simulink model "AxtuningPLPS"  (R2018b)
settings: Solver=VariableStepAuto  StartTime=0.0  StopTime=1  RelTol=1e-3
libraries: fuzblock x18

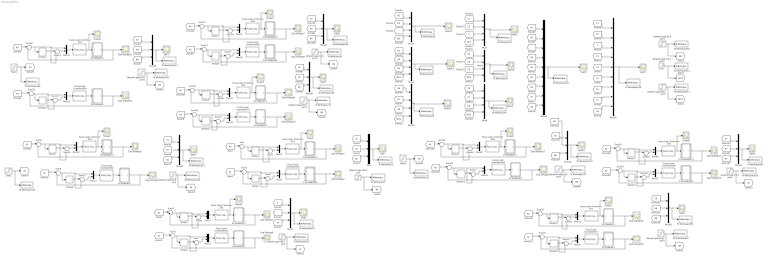
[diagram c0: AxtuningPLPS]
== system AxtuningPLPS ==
  2V EDMGAP 1 : Subsystem
  2V EDMGAP 2 : Subsystem
  2V EDMGAP 3 : Subsystem
  2V EDMGAP1 : Subsystem
  2V EDMGAP2 : Subsystem
  2V EDMGAP3 : Subsystem
  3.5V EDMGAP 1 : Subsystem
  3.5V EDMGAP 2 : Subsystem
  3.5V EDMGAP 3 : Subsystem
  3.5V EDMGAP1 : Subsystem
  3.5V EDMGAP2 : Subsystem
  3.5V EDMGAP3 : Subsystem
  5V EDMGAP 1 : Subsystem
  5V EDMGAP 2 : Subsystem
  5V EDMGAP 3 : Subsystem
  5V EDMGAP1 : Subsystem
  5V EDMGAP2 : Subsystem
  5V EDMGAP3 : Subsystem
  Delay{1..18} (18 alike) : Delay  DelayLength=1
  Fuzzy Logic Controller 3X1 : fuzblock/Fuzzy Logic  Controller  FIS=PL36  OutputSampleNumber=101  DataType=double  FuzzifiedInputs=off  RuleFiringStrengths=off  RuleOutputs=off  AggregatedOutputs=off  SimulateUsing=Interpreted execution  OutOfRangeInputValueMessage=warning  NoRuleFiredMessage=warning  EmptyOutputFuzzySetMessage=warning
  Fuzzy Logic Controller 3X2 : fuzblock/Fuzzy Logic  Controller  FIS=PL60  OutputSampleNumber=101  DataType=double  FuzzifiedInputs=off  RuleFiringStrengths=off  RuleOutputs=off  AggregatedOutputs=off  SimulateUsing=Interpreted execution  OutOfRangeInputValueMessage=warning  NoRuleFiredMessage=warning  EmptyOutputFuzzySetMessage=warning
  Fuzzy Logic Controller 3X3 : fuzblock/Fuzzy Logic  Controller  FIS=PL40  OutputSampleNumber=101  DataType=double  FuzzifiedInputs=off  RuleFiringStrengths=off  RuleOutputs=off  AggregatedOutputs=off  SimulateUsing=Interpreted execution  OutOfRangeInputValueMessage=warning  NoRuleFiredMessage=warning  EmptyOutputFuzzySetMessage=warning
  Fuzzy Logic Controller 3X4 : fuzblock/Fuzzy Logic  Controller  FIS=PL36  OutputSampleNumber=101  DataType=double  FuzzifiedInputs=off  RuleFiringStrengths=off  RuleOutputs=off  AggregatedOutputs=off  SimulateUsing=Interpreted execution  OutOfRangeInputValueMessage=warning  NoRuleFiredMessage=warning  EmptyOutputFuzzySetMessage=warning
  Fuzzy Logic Controller 3X5 : fuzblock/Fuzzy Logic  Controller  FIS=PL60  OutputSampleNumber=101  DataType=double  FuzzifiedInputs=off  RuleFiringStrengths=off  RuleOutputs=off  AggregatedOutputs=off  SimulateUsing=Interpreted execution  OutOfRangeInputValueMessage=warning  NoRuleFiredMessage=warning  EmptyOutputFuzzySetMessage=warning
  Fuzzy Logic Controller 3X6 : fuzblock/Fuzzy Logic  Controller  FIS=PL40  OutputSampleNumber=101  DataType=double  FuzzifiedInputs=off  RuleFiringStrengths=off  RuleOutputs=off  AggregatedOutputs=off  SimulateUsing=Interpreted execution  OutOfRangeInputValueMessage=warning  NoRuleFiredMessage=warning  EmptyOutputFuzzySetMessage=warning
  Fuzzy Logic Controller 3X7 : fuzblock/Fuzzy Logic  Controller  FIS=PL36  OutputSampleNumber=101  DataType=double  FuzzifiedInputs=off  RuleFiringStrengths=off  RuleOutputs=off  AggregatedOutputs=off  SimulateUsing=Interpreted execution  OutOfRangeInputValueMessage=warning  NoRuleFiredMessage=warning  EmptyOutputFuzzySetMessage=warning
  Fuzzy Logic Controller 3X8 : fuzblock/Fuzzy Logic  Controller  FIS=PL60  OutputSampleNumber=101  DataType=double  FuzzifiedInputs=off  RuleFiringStrengths=off  RuleOutputs=off  AggregatedOutputs=off  SimulateUsing=Interpreted execution  OutOfRangeInputValueMessage=warning  NoRuleFiredMessage=warning  EmptyOutputFuzzySetMessage=warning
  Fuzzy Logic Controller 3X9 : fuzblock/Fuzzy Logic  Controller  FIS=PL40  OutputSampleNumber=101  DataType=double  FuzzifiedInputs=off  RuleFiringStrengths=off  RuleOutputs=off  AggregatedOutputs=off  SimulateUsing=Interpreted execution  OutOfRangeInputValueMessage=warning  NoRuleFiredMessage=warning  EmptyOutputFuzzySetMessage=warning
  Fuzzy Logic Controller5X1 : fuzblock/Fuzzy Logic  Controller  FIS=PS25  OutputSampleNumber=101  DataType=double  FuzzifiedInputs=off  RuleFiringStrengths=off  RuleOutputs=off  AggregatedOutputs=off  SimulateUsing=Interpreted execution  OutOfRangeInputValueMessage=warning  NoRuleFiredMessage=warning  EmptyOutputFuzzySetMessage=warning
  Fuzzy Logic Controller5X2 : fuzblock/Fuzzy Logic  Controller  FIS=PS39  OutputSampleNumber=101  DataType=double  FuzzifiedInputs=off  RuleFiringStrengths=off  RuleOutputs=off  AggregatedOutputs=off  SimulateUsing=Interpreted execution  OutOfRangeInputValueMessage=warning  NoRuleFiredMessage=warning  EmptyOutputFuzzySetMessage=warning
  Fuzzy Logic Controller5X3 : fuzblock/Fuzzy Logic  Controller  FIS=PS25  OutputSampleNumber=101  DataType=double  FuzzifiedInputs=off  RuleFiringStrengths=off  RuleOutputs=off  AggregatedOutputs=off  SimulateUsing=Interpreted execution  OutOfRangeInputValueMessage=warning  NoRuleFiredMessage=warning  EmptyOutputFuzzySetMessage=warning
  Fuzzy Logic Controller5X4 : fuzblock/Fuzzy Logic  Controller  FIS=PS39  OutputSampleNumber=101  DataType=double  FuzzifiedInputs=off  RuleFiringStrengths=off  RuleOutputs=off  AggregatedOutputs=off  SimulateUsing=Interpreted execution  OutOfRangeInputValueMessage=warning  NoRuleFiredMessage=warning  EmptyOutputFuzzySetMessage=warning
  Fuzzy Logic Controller5X5 : fuzblock/Fuzzy Logic  Controller  FIS=PS35  OutputSampleNumber=101  DataType=double  FuzzifiedInputs=off  RuleFiringStrengths=off  RuleOutputs=off  AggregatedOutputs=off  SimulateUsing=Interpreted execution  OutOfRangeInputValueMessage=warning  NoRuleFiredMessage=warning  EmptyOutputFuzzySetMessage=warning
  Fuzzy Logic Controller5X6 : fuzblock/Fuzzy Logic  Controller  FIS=PS35  OutputSampleNumber=101  DataType=double  FuzzifiedInputs=off  RuleFiringStrengths=off  RuleOutputs=off  AggregatedOutputs=off  SimulateUsing=Interpreted execution  OutOfRangeInputValueMessage=warning  NoRuleFiredMessage=warning  EmptyOutputFuzzySetMessage=warning
  Fuzzy Logic Controller5X7 : fuzblock/Fuzzy Logic  Controller  FIS=PS25  OutputSampleNumber=101  DataType=double  FuzzifiedInputs=off  RuleFiringStrengths=off  RuleOutputs=off  AggregatedOutputs=off  SimulateUsing=Interpreted execution  OutOfRangeInputValueMessage=warning  NoRuleFiredMessage=warning  EmptyOutputFuzzySetMessage=warning
  Fuzzy Logic Controller5X8 : fuzblock/Fuzzy Logic  Controller  FIS=PS39  OutputSampleNumber=101  DataType=double  FuzzifiedInputs=off  RuleFiringStrengths=off  RuleOutputs=off  AggregatedOutputs=off  SimulateUsing=Interpreted execution  OutOfRangeInputValueMessage=warning  NoRuleFiredMessage=warning  EmptyOutputFuzzySetMessage=warning
  Fuzzy Logic Controller5X9 : fuzblock/Fuzzy Logic  Controller  FIS=PS35  OutputSampleNumber=101  DataType=double  FuzzifiedInputs=off  RuleFiringStrengths=off  RuleOutputs=off  AggregatedOutputs=off  SimulateUsing=Interpreted execution  OutOfRangeInputValueMessage=warning  NoRuleFiredMessage=warning  EmptyOutputFuzzySetMessage=warning
  GAP{,1..16} (17 alike) : Scope
  Gap Voltage{1..18} (18 alike) : Scope
  Mux{,6,12,26,30,40,44,48,58} (9 alike) : Mux  Inputs=3
  Mux{1,5,7,11,13,17,27,29,31,35,39,41,45,47,49,53,57,59} (18 alike) : Mux  Inputs=2
  Mux{2..4,8..10} (6 alike) : Mux
  Mux18 : Mux  Inputs=9
  Mux22 : Mux  Inputs=9
  Scope{,1..8} (9 alike) : Scope
  Setpoint gap (59,3 µm){,1..3} (4 alike) : Step  Time=0  After=59.3  SampleTime=0
  Setpoint gap (84,7 µm){,1..3} (4 alike) : Step  Time=0  After=84.7  SampleTime=0
  Setpoint gap(33,8 µm){,1..3} (4 alike) : Step  Time=0  After=33.8  SampleTime=0
  Step1 : Step  Time=0  After=3.5  SampleTime=0
  Step2 : Step  Time=0  After=2  SampleTime=0
  Step3 : Step  Time=0  After=5  SampleTime=0
  Sum{,1..35} (36 alike) : Sum  Inputs=|-+
  To Workspace1 : ToWorkspace  VariableName=setpointgap  SaveFormat=Timeseries  SampleTime=-1
  To Workspace10 : ToWorkspace  VariableName=setpointgap9  SaveFormat=Timeseries  SampleTime=-1
  To Workspace11 : ToWorkspace  VariableName=setpointgap10  SaveFormat=Timeseries  SampleTime=-1
  To Workspace12 : ToWorkspace  VariableName=setpointgap1  SaveFormat=Timeseries  SampleTime=-1
  To Workspace13 : ToWorkspace  VariableName=setpointgap11  SaveFormat=Timeseries  SampleTime=-1
  To Workspace15 : ToWorkspace  VariableName=setpointgap3  SaveFormat=Timeseries  SampleTime=-1
  To Workspace2 : ToWorkspace  VariableName=setpointgap4  SaveFormat=Timeseries  SampleTime=-1
  To Workspace22 : ToWorkspace  VariableName=gap10  SaveFormat=Timeseries  SampleTime=-1
  To Workspace23 : ToWorkspace  VariableName=setpointgap2  SaveFormat=Timeseries  SampleTime=-1
  To Workspace28 : ToWorkspace  VariableName=setpoint2  SaveFormat=Timeseries  SampleTime=-1
  To Workspace3 : ToWorkspace  VariableName=gap  SaveFormat=Timeseries  SampleTime=-1
  To Workspace33 : ToWorkspace  VariableName=gap1  SaveFormat=Timeseries  SampleTime=-1
  To Workspace39 : ToWorkspace  VariableName=gap18  SaveFormat=Timeseries  SampleTime=-1
  To Workspace4 : ToWorkspace  VariableName=gap2  SaveFormat=Timeseries  SampleTime=-1
  To Workspace43 : ToWorkspace  VariableName=gap19  SaveFormat=Timeseries  SampleTime=-1
  To Workspace44 : ToWorkspace  VariableName=gap11  SaveFormat=Timeseries  SampleTime=-1
  To Workspace45 : ToWorkspace  VariableName=setpointgap5  SaveFormat=Timeseries  SampleTime=-1
  To Workspace48 : ToWorkspace  VariableName=setpoint  SaveFormat=Timeseries  SampleTime=-1
  To Workspace5 : ToWorkspace  VariableName=gap3  SaveFormat=Timeseries  SampleTime=-1
  To Workspace53 : ToWorkspace  VariableName=gap12  SaveFormat=Timeseries  SampleTime=-1
  To Workspace58 : ToWorkspace  VariableName=gap13  SaveFormat=Timeseries  SampleTime=-1
  To Workspace59 : ToWorkspace  VariableName=setpointgap6  SaveFormat=Timeseries  SampleTime=-1
  To Workspace6 : ToWorkspace  VariableName=gap4  SaveFormat=Timeseries  SampleTime=-1
  To Workspace62 : ToWorkspace  VariableName=setpointgap7  SaveFormat=Timeseries  SampleTime=-1
  To Workspace69 : ToWorkspace  VariableName=gap14  SaveFormat=Timeseries  SampleTime=-1
  To Workspace7 : ToWorkspace  VariableName=gap5  SaveFormat=Timeseries  SampleTime=-1
  To Workspace70 : ToWorkspace  VariableName=setpointgap8  SaveFormat=Timeseries  SampleTime=-1
  To Workspace73 : ToWorkspace  VariableName=setpoint1  SaveFormat=Timeseries  SampleTime=-1
  To Workspace78 : ToWorkspace  VariableName=gap15  SaveFormat=Timeseries  SampleTime=-1
  To Workspace8 : ToWorkspace  VariableName=gap6  SaveFormat=Timeseries  SampleTime=-1
  To Workspace83 : ToWorkspace  VariableName=gap16  SaveFormat=Timeseries  SampleTime=-1
  To Workspace9 : ToWorkspace  VariableName=gap9  SaveFormat=Timeseries  SampleTime=-1
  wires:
  [N2] -> Mux/3
  Sum2/1 -> Mux1/2
  Mux5/1 -> Fuzzy Logic Controller5X5/1
  Delay2/1 -> Sum3/1
  [H2] -> Mux/2
  Mux/1 -> To Workspace9/1, GAP/1
  Sum/1 -> Delay1/1, Sum2/2, Mux1/1
  Delay1/1 -> Sum2/1
  Mux1/1 -> Fuzzy Logic Controller 3X3/1
  Fuzzy Logic Controller 3X3/1 -> Scope/1, 3.5V EDMGAP 1/1(In1)
  [A1] -> Sum1/1
  Sum1/1 -> Delay2/1, Sum3/2, Mux5/1
  Sum3/1 -> Mux5/2
  [C2] -> Mux/1
  [A1] -> Sum/1
  3.5V EDMGAP2/1(Out1) -> Gap Voltage2/1, Sum1/2
  3.5V EDMGAP 1/1(Out1) -> Sum/2, Gap Voltage1/1
  Fuzzy Logic Controller5X5/1 -> 3.5V EDMGAP2/1(In1)
  2V EDMGAP3/1(Out1) -> Gap Voltage6/1, Sum9/2
  Fuzzy Logic Controller5X2/1 -> 2V EDMGAP3/1(In1)
  [H1] -> Mux12/2
  [N1] -> Mux12/3
  [C1] -> Mux12/1
  Mux12/1 -> To Workspace33/1, GAP2/1
  Sum11/1 -> Mux17/2
  Sum9/1 -> Delay6/1, Sum11/2, Mux17/1
  Mux13/1 -> Fuzzy Logic Controller 3X2/1
  Step2/1 -> To Workspace28/1, [A1]
  [A1] -> Sum9/1
  Fuzzy Logic Controller 3X2/1 -> Scope2/1, 2V EDMGAP 3/1(In1)
  Delay5/1 -> Sum10/1
  2V EDMGAP 3/1(Out1) -> Sum8/2, Gap Voltage5/1
  Delay6/1 -> Sum11/1
  Sum10/1 -> Mux13/2
  [A1] -> Sum8/1
  Sum8/1 -> Delay5/1, Sum10/2, Mux13/1
  Mux17/1 -> Fuzzy Logic Controller5X2/1
  [H3] -> Mux30/2
  Fuzzy Logic Controller5X4/1 -> 2V EDMGAP1/1(In1)
  [N3] -> Mux30/3
  Sum17/1 -> Mux39/2
  Mux35/1 -> Fuzzy Logic Controller5X4/1
  [A3] -> Sum22/1
  Sum22/1 -> Delay11/1, Sum14/2, Mux31/1
  Step1/1 -> To Workspace48/1, [A3]
  3.5V EDMGAP1/1(Out1) -> Gap Voltage8/1, Sum13/2
  [A3] -> Sum13/1
  Fuzzy Logic Controller 3X6/1 -> Scope3/1, 3.5V EDMGAP 2/1(In1)
  Delay12/1 -> Sum15/1
  Fuzzy Logic Controller 3X5/1 -> Scope5/1, 2V EDMGAP 1/1(In1)
  [H4] -> Mux26/2
  [A3] -> Sum23/1
  Sum23/1 -> Delay12/1, Sum15/2, Mux35/1
  Mux26/1 -> To Workspace58/1, GAP5/1
  [C4] -> Mux26/1
  Mux30/1 -> To Workspace53/1, GAP7/1
  2V EDMGAP1/1(Out1) -> Gap Voltage12/1, Sum23/2
  Delay11/1 -> Sum14/1
  Sum15/1 -> Mux35/2
  Delay7/1 -> Sum16/1
  Fuzzy Logic Controller5X6/1 -> 3.5V EDMGAP1/1(In1)
  [A3] -> Sum12/1
  Delay8/1 -> Sum17/1
  Mux31/1 -> Fuzzy Logic Controller 3X5/1
  Mux27/1 -> Fuzzy Logic Controller 3X6/1
  3.5V EDMGAP 2/1(Out1) -> Sum12/2, Gap Voltage7/1
  [C3] -> Mux30/1
  Sum13/1 -> Delay8/1, Sum17/2, Mux39/1
  Sum12/1 -> Delay7/1, Sum16/2, Mux27/1
  2V EDMGAP 1/1(Out1) -> Sum22/2, Gap Voltage11/1
  Sum16/1 -> Mux27/2
  Sum14/1 -> Mux31/2
  [N4] -> Mux26/3
  Mux39/1 -> Fuzzy Logic Controller5X6/1
  Setpoint gap(33,8 µm)1/1 -> [N3], To Workspace45/1
  Setpoint gap (59,3 µm)1/1 -> [N4], To Workspace2/1
  Setpoint gap(33,8 µm)/1 -> [N1], To Workspace23/1
  Setpoint gap (59,3 µm)/1 -> [N2], To Workspace1/1
  Sum4/1 -> Delay3/1, Sum6/2, Mux7/1
  Mux7/1 -> Fuzzy Logic Controller 3X1/1
  Mux6/1 -> To Workspace22/1, GAP1/1
  5V EDMGAP1/1(Out1) -> Gap Voltage4/1, Sum5/2
  Setpoint gap (84,7 µm)/1 -> [N], To Workspace12/1
  5V EDMGAP 2/1(Out1) -> Sum4/2, Gap Voltage3/1
  Mux11/1 -> Fuzzy Logic Controller5X1/1
  Delay4/1 -> Sum7/1
  Fuzzy Logic Controller 3X1/1 -> Scope1/1, 5V EDMGAP 2/1(In1)
  Fuzzy Logic Controller5X1/1 -> 5V EDMGAP1/1(In1)
  Sum7/1 -> Mux11/2
  Sum6/1 -> Mux7/2
  Sum5/1 -> Delay4/1, Sum7/2, Mux11/1
  Delay3/1 -> Sum6/1
  [A1] -> Sum5/1
  [A1] -> Sum4/1
  [C] -> Mux6/1
  [H] -> Mux6/2
  [N] -> Mux6/3
  Setpoint gap (84,7 µm)1/1 -> [N5], To Workspace15/1
  Sum20/1 -> Mux41/2
  Sum19/1 -> Delay10/1, Sum21/2, Mux29/1
  [N5] -> Mux40/3
  Sum21/1 -> Mux29/2
  [A3] -> Sum19/1
  Delay9/1 -> Sum20/1
  Fuzzy Logic Controller5X3/1 -> 5V EDMGAP2/1(In1)
  Mux41/1 -> Fuzzy Logic Controller 3X4/1
  Delay10/1 -> Sum21/1
  Mux29/1 -> Fuzzy Logic Controller5X3/1
  5V EDMGAP2/1(Out1) -> Gap Voltage10/1, Sum19/2
  Mux40/1 -> To Workspace44/1, GAP6/1
  Fuzzy Logic Controller 3X4/1 -> Scope4/1, 5V EDMGAP 1/1(In1)
  Sum18/1 -> Delay9/1, Sum20/2, Mux41/1
  [A3] -> Sum18/1
  [H5] -> Mux40/2
  5V EDMGAP 1/1(Out1) -> Sum18/2, Gap Voltage9/1
  [C5] -> Mux40/1
  [H1] -> Mux22/1
  [H2] -> Mux22/2
  [C] -> Mux18/3
  [C2] -> Mux18/2
  [C1] -> Mux18/1
  [H] -> Mux22/3
  [C5] -> Mux18/6
  [C6] -> Mux18/7
  [C7] -> Mux18/8
  [C3] -> Mux18/4
  [C4] -> Mux18/5
  [C8] -> Mux18/9
  Mux18/1 -> To Workspace39/1, GAP3/1
  [H3] -> Mux22/4
  [H4] -> Mux22/5
  [H5] -> Mux22/6
  [H6] -> Mux22/7
  [H7] -> Mux22/8
  [H8] -> Mux22/9
  Mux22/1 -> To Workspace43/1, GAP4/1
  [C1] -> Mux2/1
  Mux2/1 -> To Workspace3/1, GAP11/1
  [C2] -> Mux2/2
  [C] -> Mux2/3
  [C4] -> Mux3/2
  [C3] -> Mux3/1
  Mux3/1 -> To Workspace4/1, GAP12/1
  [C5] -> Mux3/3
  [C8] -> Mux4/3
  [C7] -> Mux4/2
  Mux4/1 -> To Workspace5/1, GAP13/1
  [C6] -> Mux4/1
  Mux8/1 -> To Workspace6/1, GAP14/1
  [H] -> Mux8/3
  [H2] -> Mux8/2
  [H1] -> Mux8/1
  Mux9/1 -> To Workspace7/1, GAP15/1
  [H4] -> Mux9/2
  [H3] -> Mux9/1
  [H5] -> Mux9/3
  Mux10/1 -> To Workspace8/1, GAP16/1
  [H6] -> Mux10/1
  [H7] -> Mux10/2
  [H8] -> Mux10/3
  Fuzzy Logic Controller5X7/1 -> 5V EDMGAP3/1(In1)
  [C8] -> Mux58/1
  [H8] -> Mux58/2
  5V EDMGAP 3/1(Out1) -> Sum30/2, Gap Voltage15/1
  Mux59/1 -> Fuzzy Logic Controller 3X7/1
  [A2] -> Sum31/1
  Sum30/1 -> Delay15/1, Sum32/2, Mux59/1
  Setpoint gap (84,7 µm)2/1 -> [N8], To Workspace62/1
  5V EDMGAP3/1(Out1) -> Gap Voltage16/1, Sum31/2
  Sum32/1 -> Mux59/2
  Sum33/1 -> Mux47/2
  [A2] -> Sum30/1
  Sum31/1 -> Delay16/1, Sum33/2, Mux47/1
  [N8] -> Mux58/3
  2V EDMGAP 2/1(Out1) -> Sum34/2, Gap Voltage17/1
  Sum24/1 -> Delay13/1, Sum28/2, Mux45/1
  Delay15/1 -> Sum32/1
  [C6] -> Mux48/1
  3.5V EDMGAP 3/1(Out1) -> Sum24/2, Gap Voltage13/1
  Mux45/1 -> Fuzzy Logic Controller 3X9/1
  Fuzzy Logic Controller 3X7/1 -> Scope7/1, 5V EDMGAP 3/1(In1)
  [A2] -> Sum24/1
  Mux49/1 -> Fuzzy Logic Controller 3X8/1
  Delay14/1 -> Sum29/1
  Delay13/1 -> Sum28/1
  Fuzzy Logic Controller5X9/1 -> 3.5V EDMGAP3/1(In1)
  [C7] -> Mux44/1
  Mux48/1 -> To Workspace78/1, GAP10/1
  [H7] -> Mux44/2
  Fuzzy Logic Controller 3X8/1 -> Scope8/1, 2V EDMGAP 2/1(In1)
  Sum25/1 -> Delay14/1, Sum29/2, Mux57/1
  Fuzzy Logic Controller 3X9/1 -> Scope6/1, 3.5V EDMGAP 3/1(In1)
  [A2] -> Sum25/1
  Sum35/1 -> Delay18/1, Sum27/2, Mux53/1
  Mux44/1 -> To Workspace83/1, GAP8/1
  3.5V EDMGAP3/1(Out1) -> Gap Voltage14/1, Sum25/2
  Delay17/1 -> Sum26/1
  2V EDMGAP2/1(Out1) -> Gap Voltage18/1, Sum35/2
  Sum34/1 -> Delay17/1, Sum26/2, Mux49/1
  Mux53/1 -> Fuzzy Logic Controller5X8/1
  [H6] -> Mux48/2
  Sum29/1 -> Mux57/2
  Fuzzy Logic Controller5X8/1 -> 2V EDMGAP2/1(In1)
  [N7] -> Mux44/3
  [A2] -> Sum34/1
  Sum28/1 -> Mux45/2
  Sum26/1 -> Mux49/2
  [A2] -> Sum35/1
  Delay16/1 -> Sum33/1
  Mux47/1 -> Fuzzy Logic Controller5X7/1
  Step3/1 -> To Workspace73/1, [A2]
  Mux58/1 -> To Workspace69/1, GAP9/1
  Delay18/1 -> Sum27/1
  Sum27/1 -> Mux53/2
  [N6] -> Mux48/3
  Setpoint gap(33,8 µm)2/1 -> [N6], To Workspace70/1
  Mux57/1 -> Fuzzy Logic Controller5X9/1
  Setpoint gap (59,3 µm)2/1 -> [N7], To Workspace59/1
  Setpoint gap (59,3 µm)3/1 -> [SET1], To Workspace13/1
  Setpoint gap (84,7 µm)3/1 -> [SET2], To Workspace11/1
  Setpoint gap(33,8 µm)3/1 -> [SET], To Workspace10/1
  [SET] -> Mux2/4
  [SET] -> Mux8/4
  [SET1] -> Mux9/4
  [SET1] -> Mux3/4
  [SET2] -> Mux10/4
  [SET2] -> Mux4/4

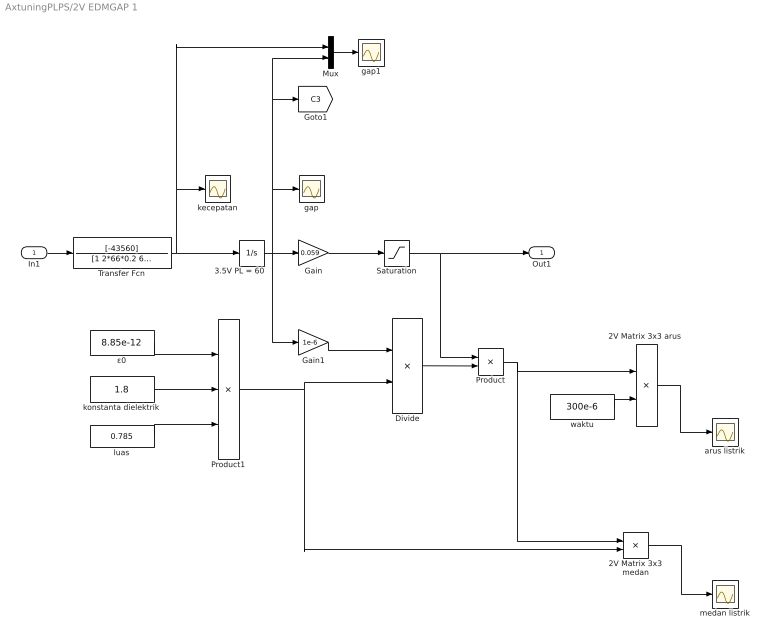
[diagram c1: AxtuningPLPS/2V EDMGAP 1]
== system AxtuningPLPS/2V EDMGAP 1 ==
  In1 : Inport
  "2V Matrix 3x3 arus " : Product  Inputs=*/
  2V Matrix 3x3 medan : Product  Inputs=*/
  3.5V PL = 60 : Integrator  InitialCondition=225
  Divide : Product  Inputs=/*
  Gain : Gain  Gain=0.059
  Gain1 : Gain  Gain=1e-6
  Mux : Mux  Inputs=2
  Product : Product
  Product1 : Product  Inputs=3
  Saturation : Saturate  UpperLimit=10  LowerLimit=0
  Transfer Fcn : TransferFcn  Numerator=[-43560]  Denominator=[1 2*66*0.2 66^2]
  arus listrik : Scope
  gap : Scope
  gap1 : Scope
  kecepatan : Scope
  konstanta dielektrik : Constant  Value=1.8
  luas : Constant  Value=0.785
  medan listrik : Scope
  waktu : Constant  Value=300e-6
  ε0 : Constant  Value=8.85e-12
  Out1 : Outport
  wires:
  3.5V PL = 60/1 -> Gain1/1, Mux/2, [C3], gap/1, Gain/1
  In1/1 -> Transfer Fcn/1
  Gain1/1 -> Divide/1
  Product1/1 -> 2V Matrix 3x3 medan/2, Divide/2
  ε0/1 -> Product1/1
  konstanta dielektrik/1 -> Product1/2
  luas/1 -> Product1/3
  Divide/1 -> Product/2
  Product/1 -> 2V Matrix 3x3 medan/1, "2V Matrix 3x3 arus "/1
  waktu/1 -> "2V Matrix 3x3 arus "/2
  "2V Matrix 3x3 arus "/1 -> arus listrik/1
  2V Matrix 3x3 medan/1 -> medan listrik/1
  Mux/1 -> gap1/1
  Transfer Fcn/1 -> Mux/1, kecepatan/1, 3.5V PL = 60/1
  Saturation/1 -> Product/1, Out1/1
  Gain/1 -> Saturation/1

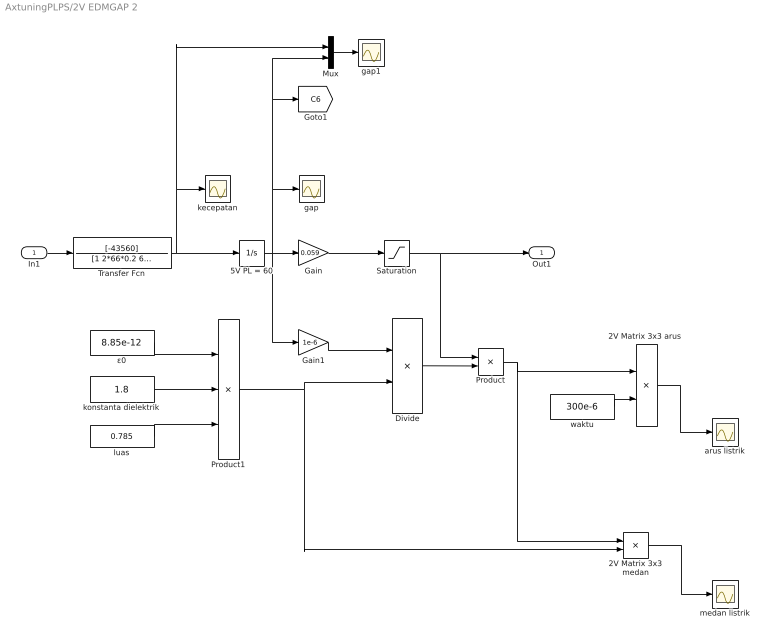
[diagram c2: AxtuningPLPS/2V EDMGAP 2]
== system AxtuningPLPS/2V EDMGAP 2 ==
  In1 : Inport
  "2V Matrix 3x3 arus " : Product  Inputs=*/
  2V Matrix 3x3 medan : Product  Inputs=*/
  5V PL = 60 : Integrator  InitialCondition=225
  Divide : Product  Inputs=/*
  Gain : Gain  Gain=0.059
  Gain1 : Gain  Gain=1e-6
  Mux : Mux  Inputs=2
  Product : Product
  Product1 : Product  Inputs=3
  Saturation : Saturate  UpperLimit=10  LowerLimit=0
  Transfer Fcn : TransferFcn  Numerator=[-43560]  Denominator=[1 2*66*0.2 66^2]
  arus listrik : Scope
  gap : Scope
  gap1 : Scope
  kecepatan : Scope
  konstanta dielektrik : Constant  Value=1.8
  luas : Constant  Value=0.785
  medan listrik : Scope
  waktu : Constant  Value=300e-6
  ε0 : Constant  Value=8.85e-12
  Out1 : Outport
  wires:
  5V PL = 60/1 -> Gain1/1, Mux/2, [C6], gap/1, Gain/1
  In1/1 -> Transfer Fcn/1
  Gain1/1 -> Divide/1
  Product1/1 -> 2V Matrix 3x3 medan/2, Divide/2
  ε0/1 -> Product1/1
  konstanta dielektrik/1 -> Product1/2
  luas/1 -> Product1/3
  Divide/1 -> Product/2
  Product/1 -> 2V Matrix 3x3 medan/1, "2V Matrix 3x3 arus "/1
  waktu/1 -> "2V Matrix 3x3 arus "/2
  "2V Matrix 3x3 arus "/1 -> arus listrik/1
  2V Matrix 3x3 medan/1 -> medan listrik/1
  Mux/1 -> gap1/1
  Transfer Fcn/1 -> Mux/1, kecepatan/1, 5V PL = 60/1
  Saturation/1 -> Product/1, Out1/1
  Gain/1 -> Saturation/1

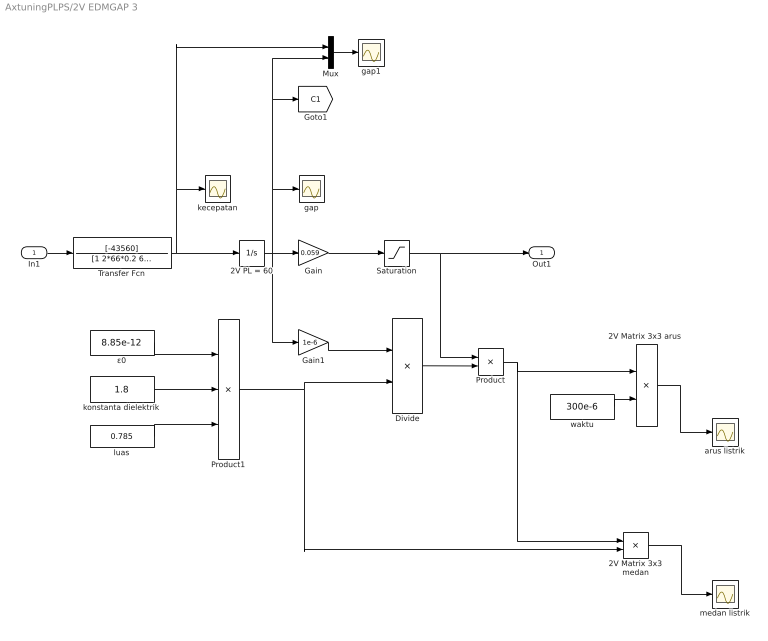
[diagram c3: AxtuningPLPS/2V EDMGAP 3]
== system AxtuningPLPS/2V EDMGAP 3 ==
  In1 : Inport
  "2V Matrix 3x3 arus " : Product  Inputs=*/
  2V Matrix 3x3 medan : Product  Inputs=*/
  2V PL = 60 : Integrator  InitialCondition=225
  Divide : Product  Inputs=/*
  Gain : Gain  Gain=0.059
  Gain1 : Gain  Gain=1e-6
  Mux : Mux  Inputs=2
  Product : Product
  Product1 : Product  Inputs=3
  Saturation : Saturate  UpperLimit=10  LowerLimit=0
  Transfer Fcn : TransferFcn  Numerator=[-43560]  Denominator=[1 2*66*0.2 66^2]
  arus listrik : Scope
  gap : Scope
  gap1 : Scope
  kecepatan : Scope
  konstanta dielektrik : Constant  Value=1.8
  luas : Constant  Value=0.785
  medan listrik : Scope
  waktu : Constant  Value=300e-6
  ε0 : Constant  Value=8.85e-12
  Out1 : Outport
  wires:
  2V PL = 60/1 -> Gain1/1, Mux/2, [C1], gap/1, Gain/1
  In1/1 -> Transfer Fcn/1
  Gain1/1 -> Divide/1
  Product1/1 -> 2V Matrix 3x3 medan/2, Divide/2
  ε0/1 -> Product1/1
  konstanta dielektrik/1 -> Product1/2
  luas/1 -> Product1/3
  Divide/1 -> Product/2
  Product/1 -> 2V Matrix 3x3 medan/1, "2V Matrix 3x3 arus "/1
  waktu/1 -> "2V Matrix 3x3 arus "/2
  "2V Matrix 3x3 arus "/1 -> arus listrik/1
  2V Matrix 3x3 medan/1 -> medan listrik/1
  Mux/1 -> gap1/1
  Transfer Fcn/1 -> Mux/1, kecepatan/1, 2V PL = 60/1
  Saturation/1 -> Product/1, Out1/1
  Gain/1 -> Saturation/1

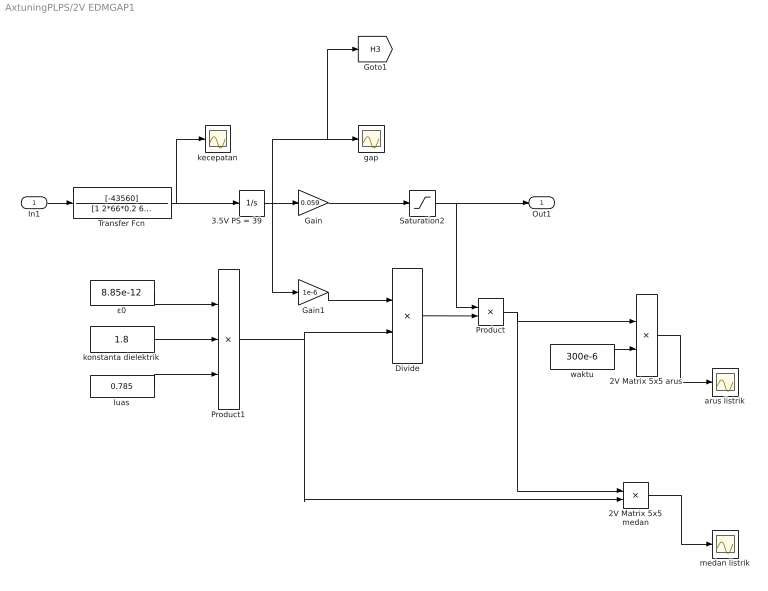
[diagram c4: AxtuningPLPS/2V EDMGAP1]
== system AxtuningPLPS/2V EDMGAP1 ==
  In1 : Inport
  2V Matrix 5x5 arus : Product  Inputs=*/
  2V Matrix 5x5 medan : Product  Inputs=*/
  "3.5V PS = 39 " : Integrator  InitialCondition=225
  Divide : Product  Inputs=/*
  Gain : Gain  Gain=0.059
  Gain1 : Gain  Gain=1e-6
  Product : Product
  Product1 : Product  Inputs=3
  Saturation2 : Saturate  UpperLimit=10  LowerLimit=0
  Transfer Fcn : TransferFcn  Numerator=[-43560]  Denominator=[1 2*66*0.2 66^2]
  arus listrik : Scope
  gap : Scope
  kecepatan : Scope
  konstanta dielektrik : Constant  Value=1.8
  luas : Constant  Value=0.785
  medan listrik : Scope
  waktu : Constant  Value=300e-6
  ε0 : Constant  Value=8.85e-12
  Out1 : Outport
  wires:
  In1/1 -> Transfer Fcn/1
  Transfer Fcn/1 -> kecepatan/1, "3.5V PS = 39 "/1
  Gain1/1 -> Divide/1
  Product1/1 -> 2V Matrix 5x5 medan/2, Divide/2
  ε0/1 -> Product1/1
  konstanta dielektrik/1 -> Product1/2
  luas/1 -> Product1/3
  Divide/1 -> Product/2
  Product/1 -> 2V Matrix 5x5 medan/1, 2V Matrix 5x5 arus/1
  waktu/1 -> 2V Matrix 5x5 arus/2
  2V Matrix 5x5 arus/1 -> arus listrik/1
  2V Matrix 5x5 medan/1 -> medan listrik/1
  "3.5V PS = 39 "/1 -> [H3], gap/1, Gain1/1, Gain/1
  Saturation2/1 -> Product/1, Out1/1
  Gain/1 -> Saturation2/1

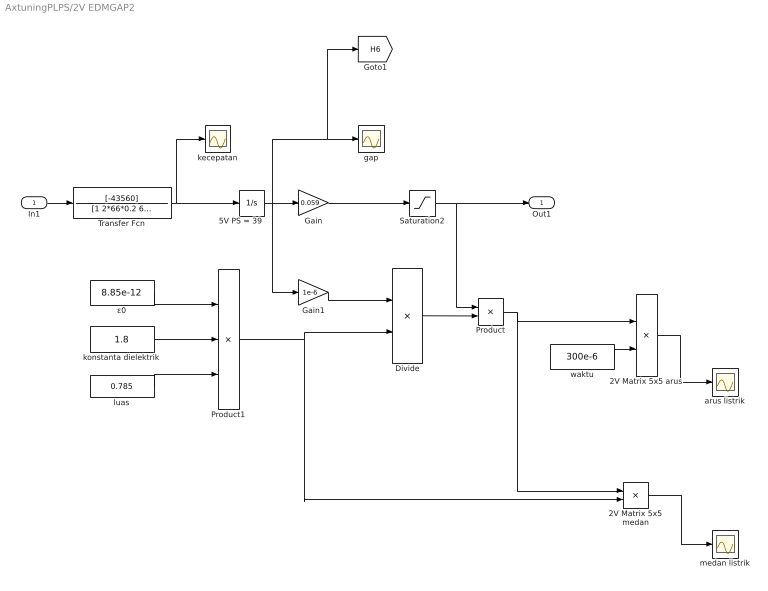
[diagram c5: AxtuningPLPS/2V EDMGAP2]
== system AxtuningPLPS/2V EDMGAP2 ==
  In1 : Inport
  2V Matrix 5x5 arus : Product  Inputs=*/
  2V Matrix 5x5 medan : Product  Inputs=*/
  "5V PS = 39 " : Integrator  InitialCondition=225
  Divide : Product  Inputs=/*
  Gain : Gain  Gain=0.059
  Gain1 : Gain  Gain=1e-6
  Product : Product
  Product1 : Product  Inputs=3
  Saturation2 : Saturate  UpperLimit=10  LowerLimit=0
  Transfer Fcn : TransferFcn  Numerator=[-43560]  Denominator=[1 2*66*0.2 66^2]
  arus listrik : Scope
  gap : Scope
  kecepatan : Scope
  konstanta dielektrik : Constant  Value=1.8
  luas : Constant  Value=0.785
  medan listrik : Scope
  waktu : Constant  Value=300e-6
  ε0 : Constant  Value=8.85e-12
  Out1 : Outport
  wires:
  In1/1 -> Transfer Fcn/1
  Transfer Fcn/1 -> kecepatan/1, "5V PS = 39 "/1
  Gain1/1 -> Divide/1
  Product1/1 -> 2V Matrix 5x5 medan/2, Divide/2
  ε0/1 -> Product1/1
  konstanta dielektrik/1 -> Product1/2
  luas/1 -> Product1/3
  Divide/1 -> Product/2
  Product/1 -> 2V Matrix 5x5 medan/1, 2V Matrix 5x5 arus/1
  waktu/1 -> 2V Matrix 5x5 arus/2
  2V Matrix 5x5 arus/1 -> arus listrik/1
  2V Matrix 5x5 medan/1 -> medan listrik/1
  "5V PS = 39 "/1 -> [H6], gap/1, Gain1/1, Gain/1
  Saturation2/1 -> Product/1, Out1/1
  Gain/1 -> Saturation2/1

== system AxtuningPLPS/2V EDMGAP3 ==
  In1 : Inport
  2V Matrix 5x5 arus : Product  Inputs=*/
  2V Matrix 5x5 medan : Product  Inputs=*/
  "2V PS = 39 " : Integrator  InitialCondition=225
  Divide : Product  Inputs=/*
  Gain : Gain  Gain=0.059
  Gain1 : Gain  Gain=1e-6
  Product : Product
  Product1 : Product  Inputs=3
  Saturation2 : Saturate  UpperLimit=10  LowerLimit=0
  Transfer Fcn : TransferFcn  Numerator=[-43560]  Denominator=[1 2*66*0.2 66^2]
  arus listrik : Scope
  gap : Scope
  kecepatan : Scope
  konstanta dielektrik : Constant  Value=1.8
  luas : Constant  Value=0.785
  medan listrik : Scope
  waktu : Constant  Value=300e-6
  ε0 : Constant  Value=8.85e-12
  Out1 : Outport
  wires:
  In1/1 -> Transfer Fcn/1
  Transfer Fcn/1 -> kecepatan/1, "2V PS = 39 "/1
  Gain1/1 -> Divide/1
  Product1/1 -> 2V Matrix 5x5 medan/2, Divide/2
  ε0/1 -> Product1/1
  konstanta dielektrik/1 -> Product1/2
  luas/1 -> Product1/3
  Divide/1 -> Product/2
  Product/1 -> 2V Matrix 5x5 medan/1, 2V Matrix 5x5 arus/1
  waktu/1 -> 2V Matrix 5x5 arus/2
  2V Matrix 5x5 arus/1 -> arus listrik/1
  2V Matrix 5x5 medan/1 -> medan listrik/1
  "2V PS = 39 "/1 -> [H1], gap/1, Gain1/1, Gain/1
  Saturation2/1 -> Product/1, Out1/1
  Gain/1 -> Saturation2/1

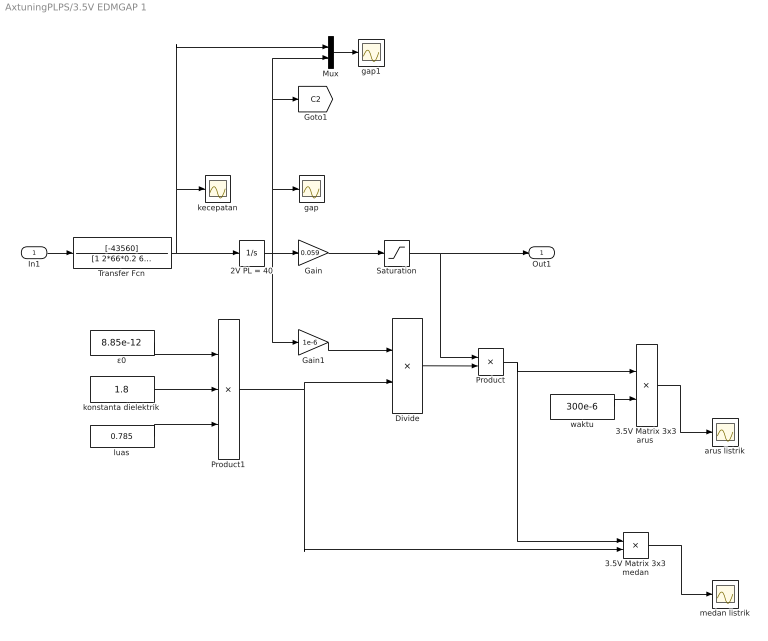
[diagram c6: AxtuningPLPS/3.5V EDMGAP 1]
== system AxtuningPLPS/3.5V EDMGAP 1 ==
  In1 : Inport
  2V PL = 40 : Integrator  InitialCondition=225
  "3.5V Matrix 3x3 arus " : Product  Inputs=*/
  3.5V Matrix 3x3 medan : Product  Inputs=*/
  Divide : Product  Inputs=/*
  Gain : Gain  Gain=0.059
  Gain1 : Gain  Gain=1e-6
  Mux : Mux  Inputs=2
  Product : Product
  Product1 : Product  Inputs=3
  Saturation : Saturate  UpperLimit=10  LowerLimit=0
  Transfer Fcn : TransferFcn  Numerator=[-43560]  Denominator=[1 2*66*0.2 66^2]
  arus listrik : Scope
  gap : Scope
  gap1 : Scope
  kecepatan : Scope
  konstanta dielektrik : Constant  Value=1.8
  luas : Constant  Value=0.785
  medan listrik : Scope
  waktu : Constant  Value=300e-6
  ε0 : Constant  Value=8.85e-12
  Out1 : Outport
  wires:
  2V PL = 40/1 -> Gain1/1, Mux/2, [C2], gap/1, Gain/1
  In1/1 -> Transfer Fcn/1
  Gain1/1 -> Divide/1
  Product1/1 -> 3.5V Matrix 3x3 medan/2, Divide/2
  ε0/1 -> Product1/1
  konstanta dielektrik/1 -> Product1/2
  luas/1 -> Product1/3
  Divide/1 -> Product/2
  Product/1 -> 3.5V Matrix 3x3 medan/1, "3.5V Matrix 3x3 arus "/1
  waktu/1 -> "3.5V Matrix 3x3 arus "/2
  "3.5V Matrix 3x3 arus "/1 -> arus listrik/1
  3.5V Matrix 3x3 medan/1 -> medan listrik/1
  Mux/1 -> gap1/1
  Transfer Fcn/1 -> Mux/1, kecepatan/1, 2V PL = 40/1
  Saturation/1 -> Product/1, Out1/1
  Gain/1 -> Saturation/1

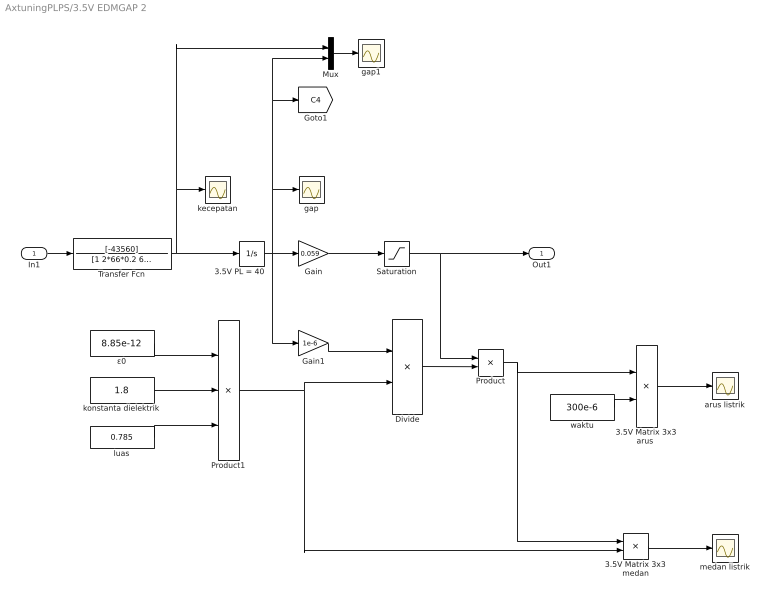
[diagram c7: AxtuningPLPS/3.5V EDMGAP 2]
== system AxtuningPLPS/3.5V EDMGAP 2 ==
  In1 : Inport
  "3.5V Matrix 3x3 arus " : Product  Inputs=*/
  3.5V Matrix 3x3 medan : Product  Inputs=*/
  3.5V PL = 40 : Integrator  InitialCondition=225
  Divide : Product  Inputs=/*
  Gain : Gain  Gain=0.059
  Gain1 : Gain  Gain=1e-6
  Mux : Mux  Inputs=2
  Product : Product
  Product1 : Product  Inputs=3
  Saturation : Saturate  UpperLimit=10  LowerLimit=0
  Transfer Fcn : TransferFcn  Numerator=[-43560]  Denominator=[1 2*66*0.2 66^2]
  arus listrik : Scope
  gap : Scope
  gap1 : Scope
  kecepatan : Scope
  konstanta dielektrik : Constant  Value=1.8
  luas : Constant  Value=0.785
  medan listrik : Scope
  waktu : Constant  Value=300e-6
  ε0 : Constant  Value=8.85e-12
  Out1 : Outport
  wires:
  3.5V PL = 40/1 -> Gain1/1, Mux/2, [C4], gap/1, Gain/1
  In1/1 -> Transfer Fcn/1
  Gain1/1 -> Divide/1
  Product1/1 -> 3.5V Matrix 3x3 medan/2, Divide/2
  ε0/1 -> Product1/1
  konstanta dielektrik/1 -> Product1/2
  luas/1 -> Product1/3
  Divide/1 -> Product/2
  Product/1 -> 3.5V Matrix 3x3 medan/1, "3.5V Matrix 3x3 arus "/1
  waktu/1 -> "3.5V Matrix 3x3 arus "/2
  "3.5V Matrix 3x3 arus "/1 -> arus listrik/1
  3.5V Matrix 3x3 medan/1 -> medan listrik/1
  Mux/1 -> gap1/1
  Transfer Fcn/1 -> Mux/1, kecepatan/1, 3.5V PL = 40/1
  Saturation/1 -> Product/1, Out1/1
  Gain/1 -> Saturation/1

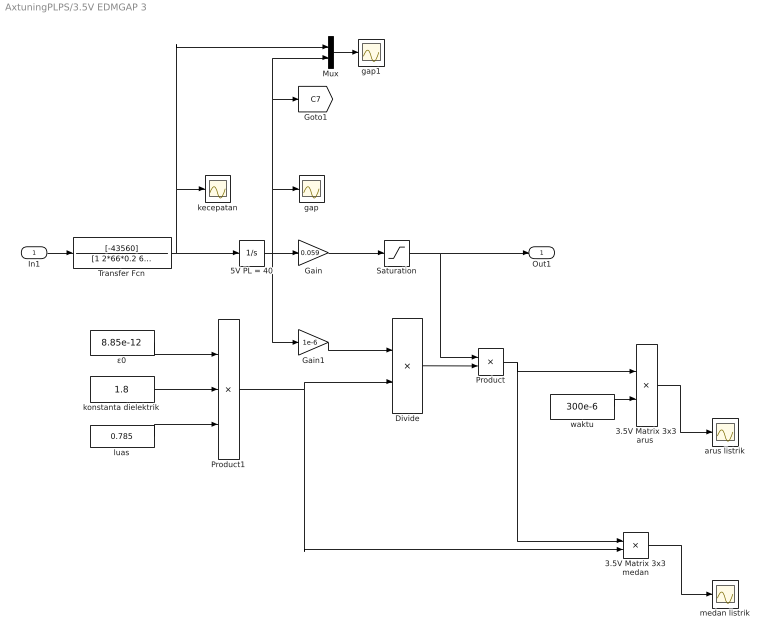
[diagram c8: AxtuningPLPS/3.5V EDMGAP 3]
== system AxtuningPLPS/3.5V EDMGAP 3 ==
  In1 : Inport
  "3.5V Matrix 3x3 arus " : Product  Inputs=*/
  3.5V Matrix 3x3 medan : Product  Inputs=*/
  5V PL = 40 : Integrator  InitialCondition=225
  Divide : Product  Inputs=/*
  Gain : Gain  Gain=0.059
  Gain1 : Gain  Gain=1e-6
  Mux : Mux  Inputs=2
  Product : Product
  Product1 : Product  Inputs=3
  Saturation : Saturate  UpperLimit=10  LowerLimit=0
  Transfer Fcn : TransferFcn  Numerator=[-43560]  Denominator=[1 2*66*0.2 66^2]
  arus listrik : Scope
  gap : Scope
  gap1 : Scope
  kecepatan : Scope
  konstanta dielektrik : Constant  Value=1.8
  luas : Constant  Value=0.785
  medan listrik : Scope
  waktu : Constant  Value=300e-6
  ε0 : Constant  Value=8.85e-12
  Out1 : Outport
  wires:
  5V PL = 40/1 -> Gain1/1, Mux/2, [C7], gap/1, Gain/1
  In1/1 -> Transfer Fcn/1
  Gain1/1 -> Divide/1
  Product1/1 -> 3.5V Matrix 3x3 medan/2, Divide/2
  ε0/1 -> Product1/1
  konstanta dielektrik/1 -> Product1/2
  luas/1 -> Product1/3
  Divide/1 -> Product/2
  Product/1 -> 3.5V Matrix 3x3 medan/1, "3.5V Matrix 3x3 arus "/1
  waktu/1 -> "3.5V Matrix 3x3 arus "/2
  "3.5V Matrix 3x3 arus "/1 -> arus listrik/1
  3.5V Matrix 3x3 medan/1 -> medan listrik/1
  Mux/1 -> gap1/1
  Transfer Fcn/1 -> Mux/1, kecepatan/1, 5V PL = 40/1
  Saturation/1 -> Product/1, Out1/1
  Gain/1 -> Saturation/1

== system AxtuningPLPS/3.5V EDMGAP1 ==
  In1 : Inport
  3.5V Matrix 5x5 arus : Product  Inputs=*/
  3.5V Matrix 5x5 medan : Product  Inputs=*/
  "3.5V PS = 35  " : Integrator  InitialCondition=225
  Divide : Product  Inputs=/*
  Gain : Gain  Gain=0.059
  Gain1 : Gain  Gain=1e-6
  Product : Product
  Product1 : Product  Inputs=3
  Saturation2 : Saturate  UpperLimit=10  LowerLimit=0
  Transfer Fcn : TransferFcn  Numerator=[-43560]  Denominator=[1 2*66*0.2 66^2]
  arus listrik : Scope
  gap : Scope
  kecepatan : Scope
  konstanta dielektrik : Constant  Value=1.8
  luas : Constant  Value=0.785
  medan listrik : Scope
  waktu : Constant  Value=300e-6
  ε0 : Constant  Value=8.85e-12
  Out1 : Outport
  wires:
  In1/1 -> Transfer Fcn/1
  Transfer Fcn/1 -> kecepatan/1, "3.5V PS = 35  "/1
  Gain1/1 -> Divide/1
  Product1/1 -> 3.5V Matrix 5x5 medan/2, Divide/2
  ε0/1 -> Product1/1
  konstanta dielektrik/1 -> Product1/2
  luas/1 -> Product1/3
  Divide/1 -> Product/2
  Product/1 -> 3.5V Matrix 5x5 medan/1, 3.5V Matrix 5x5 arus/1
  waktu/1 -> 3.5V Matrix 5x5 arus/2
  3.5V Matrix 5x5 arus/1 -> arus listrik/1
  3.5V Matrix 5x5 medan/1 -> medan listrik/1
  "3.5V PS = 35  "/1 -> [H4], gap/1, Gain1/1, Gain/1
  Saturation2/1 -> Product/1, Out1/1
  Gain/1 -> Saturation2/1

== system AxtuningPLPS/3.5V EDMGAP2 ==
  In1 : Inport
  "2V PS = 35  " : Integrator  InitialCondition=225
  3.5V Matrix 5x5 arus : Product  Inputs=*/
  3.5V Matrix 5x5 medan : Product  Inputs=*/
  Divide : Product  Inputs=/*
  Gain : Gain  Gain=0.059
  Gain1 : Gain  Gain=1e-6
  Product : Product
  Product1 : Product  Inputs=3
  Saturation2 : Saturate  UpperLimit=10  LowerLimit=0
  Transfer Fcn : TransferFcn  Numerator=[-43560]  Denominator=[1 2*66*0.2 66^2]
  arus listrik : Scope
  gap : Scope
  kecepatan : Scope
  konstanta dielektrik : Constant  Value=1.8
  luas : Constant  Value=0.785
  medan listrik : Scope
  waktu : Constant  Value=300e-6
  ε0 : Constant  Value=8.85e-12
  Out1 : Outport
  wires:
  In1/1 -> Transfer Fcn/1
  Transfer Fcn/1 -> kecepatan/1, "2V PS = 35  "/1
  Gain1/1 -> Divide/1
  Product1/1 -> 3.5V Matrix 5x5 medan/2, Divide/2
  ε0/1 -> Product1/1
  konstanta dielektrik/1 -> Product1/2
  luas/1 -> Product1/3
  Divide/1 -> Product/2
  Product/1 -> 3.5V Matrix 5x5 medan/1, 3.5V Matrix 5x5 arus/1
  waktu/1 -> 3.5V Matrix 5x5 arus/2
  3.5V Matrix 5x5 arus/1 -> arus listrik/1
  3.5V Matrix 5x5 medan/1 -> medan listrik/1
  "2V PS = 35  "/1 -> [H2], gap/1, Gain1/1, Gain/1
  Saturation2/1 -> Product/1, Out1/1
  Gain/1 -> Saturation2/1

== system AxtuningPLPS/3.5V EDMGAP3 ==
  In1 : Inport
  3.5V Matrix 5x5 arus : Product  Inputs=*/
  3.5V Matrix 5x5 medan : Product  Inputs=*/
  "5V PS = 35  " : Integrator  InitialCondition=225
  Divide : Product  Inputs=/*
  Gain : Gain  Gain=0.059
  Gain1 : Gain  Gain=1e-6
  Product : Product
  Product1 : Product  Inputs=3
  Saturation2 : Saturate  UpperLimit=10  LowerLimit=0
  Transfer Fcn : TransferFcn  Numerator=[-43560]  Denominator=[1 2*66*0.2 66^2]
  arus listrik : Scope
  gap : Scope
  kecepatan : Scope
  konstanta dielektrik : Constant  Value=1.8
  luas : Constant  Value=0.785
  medan listrik : Scope
  waktu : Constant  Value=300e-6
  ε0 : Constant  Value=8.85e-12
  Out1 : Outport
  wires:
  In1/1 -> Transfer Fcn/1
  Transfer Fcn/1 -> kecepatan/1, "5V PS = 35  "/1
  Gain1/1 -> Divide/1
  Product1/1 -> 3.5V Matrix 5x5 medan/2, Divide/2
  ε0/1 -> Product1/1
  konstanta dielektrik/1 -> Product1/2
  luas/1 -> Product1/3
  Divide/1 -> Product/2
  Product/1 -> 3.5V Matrix 5x5 medan/1, 3.5V Matrix 5x5 arus/1
  waktu/1 -> 3.5V Matrix 5x5 arus/2
  3.5V Matrix 5x5 arus/1 -> arus listrik/1
  3.5V Matrix 5x5 medan/1 -> medan listrik/1
  "5V PS = 35  "/1 -> [H7], gap/1, Gain1/1, Gain/1
  Saturation2/1 -> Product/1, Out1/1
  Gain/1 -> Saturation2/1

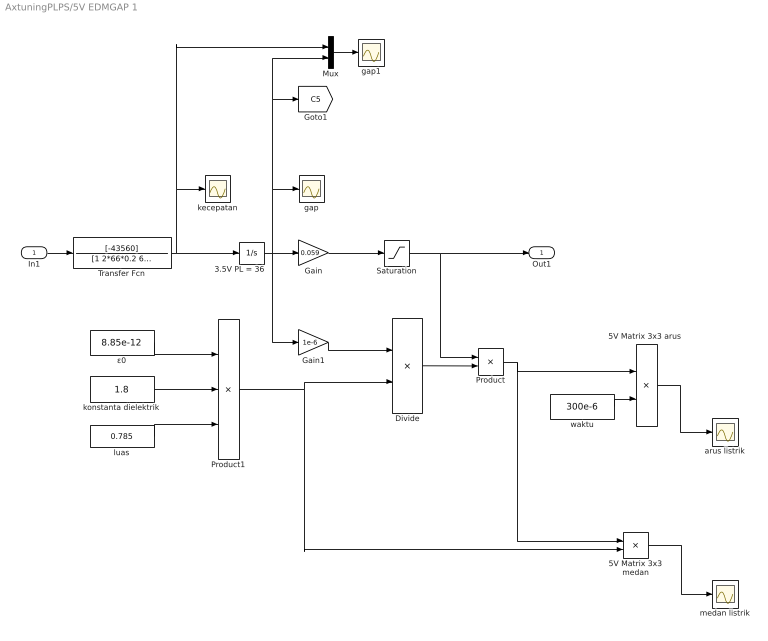
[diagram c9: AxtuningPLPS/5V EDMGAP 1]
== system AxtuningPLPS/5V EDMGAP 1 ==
  In1 : Inport
  3.5V PL = 36 : Integrator  InitialCondition=225
  "5V Matrix 3x3 arus " : Product  Inputs=*/
  5V Matrix 3x3 medan : Product  Inputs=*/
  Divide : Product  Inputs=/*
  Gain : Gain  Gain=0.059
  Gain1 : Gain  Gain=1e-6
  Mux : Mux  Inputs=2
  Product : Product
  Product1 : Product  Inputs=3
  Saturation : Saturate  UpperLimit=10  LowerLimit=0
  Transfer Fcn : TransferFcn  Numerator=[-43560]  Denominator=[1 2*66*0.2 66^2]
  arus listrik : Scope
  gap : Scope
  gap1 : Scope
  kecepatan : Scope
  konstanta dielektrik : Constant  Value=1.8
  luas : Constant  Value=0.785
  medan listrik : Scope
  waktu : Constant  Value=300e-6
  ε0 : Constant  Value=8.85e-12
  Out1 : Outport
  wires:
  3.5V PL = 36/1 -> Gain1/1, Mux/2, [C5], gap/1, Gain/1
  In1/1 -> Transfer Fcn/1
  Gain1/1 -> Divide/1
  Product1/1 -> 5V Matrix 3x3 medan/2, Divide/2
  ε0/1 -> Product1/1
  konstanta dielektrik/1 -> Product1/2
  luas/1 -> Product1/3
  Divide/1 -> Product/2
  Product/1 -> 5V Matrix 3x3 medan/1, "5V Matrix 3x3 arus "/1
  waktu/1 -> "5V Matrix 3x3 arus "/2
  "5V Matrix 3x3 arus "/1 -> arus listrik/1
  5V Matrix 3x3 medan/1 -> medan listrik/1
  Mux/1 -> gap1/1
  Transfer Fcn/1 -> Mux/1, kecepatan/1, 3.5V PL = 36/1
  Saturation/1 -> Product/1, Out1/1
  Gain/1 -> Saturation/1

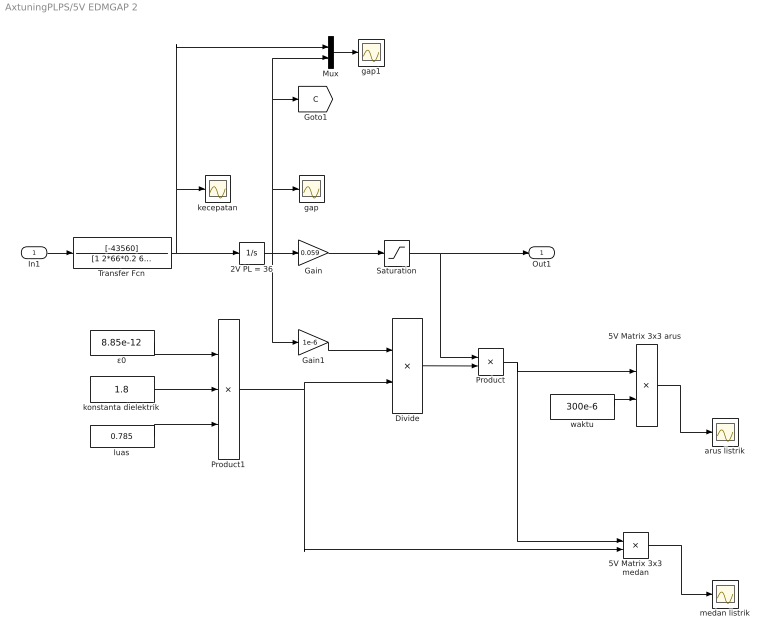
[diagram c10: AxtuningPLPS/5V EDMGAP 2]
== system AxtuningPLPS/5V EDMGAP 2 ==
  In1 : Inport
  2V PL = 36 : Integrator  InitialCondition=225
  "5V Matrix 3x3 arus " : Product  Inputs=*/
  5V Matrix 3x3 medan : Product  Inputs=*/
  Divide : Product  Inputs=/*
  Gain : Gain  Gain=0.059
  Gain1 : Gain  Gain=1e-6
  Mux : Mux  Inputs=2
  Product : Product
  Product1 : Product  Inputs=3
  Saturation : Saturate  UpperLimit=10  LowerLimit=0
  Transfer Fcn : TransferFcn  Numerator=[-43560]  Denominator=[1 2*66*0.2 66^2]
  arus listrik : Scope
  gap : Scope
  gap1 : Scope
  kecepatan : Scope
  konstanta dielektrik : Constant  Value=1.8
  luas : Constant  Value=0.785
  medan listrik : Scope
  waktu : Constant  Value=300e-6
  ε0 : Constant  Value=8.85e-12
  Out1 : Outport
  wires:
  2V PL = 36/1 -> Gain1/1, Mux/2, [C], gap/1, Gain/1
  In1/1 -> Transfer Fcn/1
  Gain1/1 -> Divide/1
  Product1/1 -> 5V Matrix 3x3 medan/2, Divide/2
  ε0/1 -> Product1/1
  konstanta dielektrik/1 -> Product1/2
  luas/1 -> Product1/3
  Divide/1 -> Product/2
  Product/1 -> 5V Matrix 3x3 medan/1, "5V Matrix 3x3 arus "/1
  waktu/1 -> "5V Matrix 3x3 arus "/2
  "5V Matrix 3x3 arus "/1 -> arus listrik/1
  5V Matrix 3x3 medan/1 -> medan listrik/1
  Mux/1 -> gap1/1
  Transfer Fcn/1 -> Mux/1, kecepatan/1, 2V PL = 36/1
  Saturation/1 -> Product/1, Out1/1
  Gain/1 -> Saturation/1

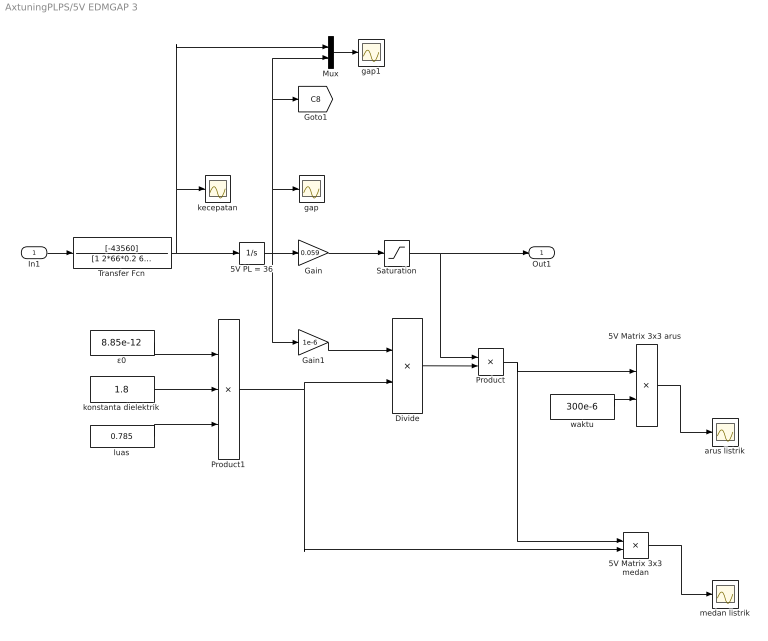
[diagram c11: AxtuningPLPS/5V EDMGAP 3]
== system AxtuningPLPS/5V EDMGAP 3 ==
  In1 : Inport
  "5V Matrix 3x3 arus " : Product  Inputs=*/
  5V Matrix 3x3 medan : Product  Inputs=*/
  5V PL = 36 : Integrator  InitialCondition=225
  Divide : Product  Inputs=/*
  Gain : Gain  Gain=0.059
  Gain1 : Gain  Gain=1e-6
  Mux : Mux  Inputs=2
  Product : Product
  Product1 : Product  Inputs=3
  Saturation : Saturate  UpperLimit=10  LowerLimit=0
  Transfer Fcn : TransferFcn  Numerator=[-43560]  Denominator=[1 2*66*0.2 66^2]
  arus listrik : Scope
  gap : Scope
  gap1 : Scope
  kecepatan : Scope
  konstanta dielektrik : Constant  Value=1.8
  luas : Constant  Value=0.785
  medan listrik : Scope
  waktu : Constant  Value=300e-6
  ε0 : Constant  Value=8.85e-12
  Out1 : Outport
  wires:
  5V PL = 36/1 -> Gain1/1, Mux/2, [C8], gap/1, Gain/1
  In1/1 -> Transfer Fcn/1
  Gain1/1 -> Divide/1
  Product1/1 -> 5V Matrix 3x3 medan/2, Divide/2
  ε0/1 -> Product1/1
  konstanta dielektrik/1 -> Product1/2
  luas/1 -> Product1/3
  Divide/1 -> Product/2
  Product/1 -> 5V Matrix 3x3 medan/1, "5V Matrix 3x3 arus "/1
  waktu/1 -> "5V Matrix 3x3 arus "/2
  "5V Matrix 3x3 arus "/1 -> arus listrik/1
  5V Matrix 3x3 medan/1 -> medan listrik/1
  Mux/1 -> gap1/1
  Transfer Fcn/1 -> Mux/1, kecepatan/1, 5V PL = 36/1
  Saturation/1 -> Product/1, Out1/1
  Gain/1 -> Saturation/1

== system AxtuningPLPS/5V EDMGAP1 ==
  In1 : Inport
  "2V PS = 25 " : Integrator  InitialCondition=225
  5V Matrix 5x5 arus : Product  Inputs=*/
  5V Matrix 5x5 medan : Product  Inputs=*/
  Divide : Product  Inputs=/*
  Gain : Gain  Gain=0.059
  Gain1 : Gain  Gain=1e-6
  Product : Product
  Product1 : Product  Inputs=3
  Saturation2 : Saturate  UpperLimit=10  LowerLimit=0
  Transfer Fcn : TransferFcn  Numerator=[-43560]  Denominator=[1 2*66*0.2 66^2]
  arus listrik : Scope
  gap : Scope
  kecepatan : Scope
  konstanta dielektrik : Constant  Value=1.8
  luas : Constant  Value=0.785
  medan listrik : Scope
  waktu : Constant  Value=300e-6
  ε0 : Constant  Value=8.85e-12
  Out1 : Outport
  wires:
  In1/1 -> Transfer Fcn/1
  Transfer Fcn/1 -> kecepatan/1, "2V PS = 25 "/1
  Gain1/1 -> Divide/1
  Product1/1 -> 5V Matrix 5x5 medan/2, Divide/2
  ε0/1 -> Product1/1
  konstanta dielektrik/1 -> Product1/2
  luas/1 -> Product1/3
  Divide/1 -> Product/2
  Product/1 -> 5V Matrix 5x5 medan/1, 5V Matrix 5x5 arus/1
  waktu/1 -> 5V Matrix 5x5 arus/2
  5V Matrix 5x5 arus/1 -> arus listrik/1
  5V Matrix 5x5 medan/1 -> medan listrik/1
  "2V PS = 25 "/1 -> [H], gap/1, Gain1/1, Gain/1
  Saturation2/1 -> Product/1, Out1/1
  Gain/1 -> Saturation2/1

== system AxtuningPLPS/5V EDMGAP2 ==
  In1 : Inport
  "3.5V PS = 25 " : Integrator  InitialCondition=225
  5V Matrix 5x5 arus : Product  Inputs=*/
  5V Matrix 5x5 medan : Product  Inputs=*/
  Divide : Product  Inputs=/*
  Gain : Gain  Gain=0.059
  Gain1 : Gain  Gain=1e-6
  Product : Product
  Product1 : Product  Inputs=3
  Saturation2 : Saturate  UpperLimit=10  LowerLimit=0
  Transfer Fcn : TransferFcn  Numerator=[-43560]  Denominator=[1 2*66*0.2 66^2]
  arus listrik : Scope
  gap : Scope
  kecepatan : Scope
  konstanta dielektrik : Constant  Value=1.8
  luas : Constant  Value=0.785
  medan listrik : Scope
  waktu : Constant  Value=300e-6
  ε0 : Constant  Value=8.85e-12
  Out1 : Outport
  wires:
  In1/1 -> Transfer Fcn/1
  Transfer Fcn/1 -> kecepatan/1, "3.5V PS = 25 "/1
  Gain1/1 -> Divide/1
  Product1/1 -> 5V Matrix 5x5 medan/2, Divide/2
  ε0/1 -> Product1/1
  konstanta dielektrik/1 -> Product1/2
  luas/1 -> Product1/3
  Divide/1 -> Product/2
  Product/1 -> 5V Matrix 5x5 medan/1, 5V Matrix 5x5 arus/1
  waktu/1 -> 5V Matrix 5x5 arus/2
  5V Matrix 5x5 arus/1 -> arus listrik/1
  5V Matrix 5x5 medan/1 -> medan listrik/1
  "3.5V PS = 25 "/1 -> [H5], gap/1, Gain1/1, Gain/1
  Saturation2/1 -> Product/1, Out1/1
  Gain/1 -> Saturation2/1

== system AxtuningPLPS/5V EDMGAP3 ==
  In1 : Inport
  5V Matrix 5x5 arus : Product  Inputs=*/
  5V Matrix 5x5 medan : Product  Inputs=*/
  "5V PS = 25 " : Integrator  InitialCondition=225
  Divide : Product  Inputs=/*
  Gain : Gain  Gain=0.059
  Gain1 : Gain  Gain=1e-6
  Product : Product
  Product1 : Product  Inputs=3
  Saturation2 : Saturate  UpperLimit=10  LowerLimit=0
  Transfer Fcn : TransferFcn  Numerator=[-43560]  Denominator=[1 2*66*0.2 66^2]
  arus listrik : Scope
  gap : Scope
  kecepatan : Scope
  konstanta dielektrik : Constant  Value=1.8
  luas : Constant  Value=0.785
  medan listrik : Scope
  waktu : Constant  Value=300e-6
  ε0 : Constant  Value=8.85e-12
  Out1 : Outport
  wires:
  In1/1 -> Transfer Fcn/1
  Transfer Fcn/1 -> kecepatan/1, "5V PS = 25 "/1
  Gain1/1 -> Divide/1
  Product1/1 -> 5V Matrix 5x5 medan/2, Divide/2
  ε0/1 -> Product1/1
  konstanta dielektrik/1 -> Product1/2
  luas/1 -> Product1/3
  Divide/1 -> Product/2
  Product/1 -> 5V Matrix 5x5 medan/1, 5V Matrix 5x5 arus/1
  waktu/1 -> 5V Matrix 5x5 arus/2
  5V Matrix 5x5 arus/1 -> arus listrik/1
  5V Matrix 5x5 medan/1 -> medan listrik/1
  "5V PS = 25 "/1 -> [H8], gap/1, Gain1/1, Gain/1
  Saturation2/1 -> Product/1, Out1/1
  Gain/1 -> Saturation2/1
